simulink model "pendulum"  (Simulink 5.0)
settings: Solver=FixedStepDiscrete  StartTime=0  StopTime=2000*Ts  FixedStep=Ts  MaxStep=0.001  RelTol=1e-3
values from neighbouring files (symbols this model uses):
  angle_K = 22/0.5    (= 44)    [pendulum_init.m]
  friction2 = 0.08    [pendulum_init.m]
  Kd = 0.00349    [pendulum_init.m]
  Kd_x = 0.2    [pendulum_init.m]
  Kp = 0.1047    [pendulum_init.m]
  Kp_x = 0.2    [pendulum_init.m]
  limit_motor = 1.1    [pendulum_init.m]
  motor_bias = -0.011    [pendulum_init.m]
  position_command = 0    [pendulum_init.m]
  POSITION_EN = 0    [pendulum_init.m]
  position_K = cm_per_rotation/400    (= 0.020375)    [pendulum_init.m]
  reset_all = 0    [pendulum_init.m]
  reset_angle = 0    [pendulum_init.m]
  reset_position = 0    [pendulum_init.m]
  reset_speed = 0    [pendulum_init.m]
  RUN = 0    [pendulum_init.m]
  slope1 = 6    [pendulum_init.m]
  slope2 = 3    [pendulum_init.m]
  speed_K = cm_per_rotation*1000/60/3    (= 45.2777777778)    [pendulum_init.m]
  trigger_voltage = 0.8    [pendulum_init.m]
undefined symbols (not defined in the file or in its folder): friction1, Ts

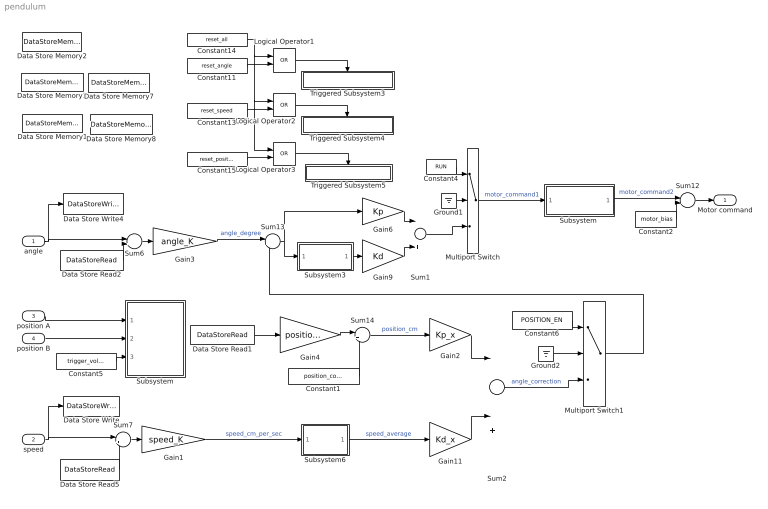
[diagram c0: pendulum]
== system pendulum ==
  angle : Inport
  speed : Inport  Port=2  ShowAdditionalParam=on
  position A : Inport  Port=3
  position B : Inport  Port=4
  Constant1 : Constant  Value=position_command  VectorParams1D=off
  Constant11 : Constant  Value=reset_angle  VectorParams1D=off
  Constant13 : Constant  Value=reset_speed  VectorParams1D=off
  Constant14 : Constant  Value=reset_all  VectorParams1D=off
  Constant15 : Constant  Value=reset_position  VectorParams1D=off
  Constant2 : Constant  Value=motor_bias  VectorParams1D=off
  Constant4 : Constant  Value=RUN  VectorParams1D=off
  Constant5 : Constant  Value=trigger_voltage  VectorParams1D=off
  Constant6 : Constant  Value=POSITION_EN  VectorParams1D=off
  Data Store Memory1 : DataStoreMemory  DataStoreName=speed_V  InitialValue=0
  Data Store Memory2 : DataStoreMemory  DataStoreName=position_count  InitialValue=0
  Data Store Memory3 : DataStoreMemory  DataStoreName=angle_V  InitialValue=0
  Data Store Memory7 : DataStoreMemory  DataStoreName=angle_V_zero  InitialValue=2.045
  Data Store Memory8 : DataStoreMemory  DataStoreName=speed_V_zero  InitialValue=0
  Data Store Read1 : DataStoreRead  DataStoreName=position_count  SampleTime=Ts
  Data Store Read2 : DataStoreRead  DataStoreName=angle_V_zero  SampleTime=Ts
  Data Store Read5 : DataStoreRead  DataStoreName=speed_V_zero  SampleTime=Ts
  Data Store Write : DataStoreWrite  DataStoreName=speed_V  SampleTime=Ts
  Data Store Write4 : DataStoreWrite  DataStoreName=angle_V  SampleTime=Ts
  Gain1 : Gain  Gain=speed_K
  Gain11 : Gain  Gain=Kd_x
  Gain2 : Gain  Gain=Kp_x
  Gain3 : Gain  Gain=angle_K
  Gain4 : Gain  Gain=position_K
  Gain6 : Gain  Gain=Kp
  Gain9 : Gain  Gain=Kd
  Ground1 : Ground
  Ground2 : Ground
  Logical Operator1 : Logic  Operator=OR  AllPortsSameDT=off
  Logical Operator2 : Logic  Operator=OR  AllPortsSameDT=off
  Logical Operator3 : Logic  Operator=OR  AllPortsSameDT=off
  Multiport Switch : MultiPortSwitch  Inputs=2  ShowAdditionalParam=on  zeroidx=on
  Multiport Switch1 : MultiPortSwitch  Inputs=2  ShowAdditionalParam=on  zeroidx=on
  Subsystem : Subsystem
  "Subsystem " : Subsystem
  Subsystem3 : Subsystem
  Subsystem6 : Subsystem
  Sum1 : Sum  Inputs=|+|||+|
  Sum{6..7,12,14} (4 alike) : Sum  Inputs=|+-
  Sum13 : Sum  Inputs=|++
  Sum2 : Sum  Inputs=||+||||||+||
  Triggered Subsystem3 : Subsystem  TreatAsAtomicUnit=on
  Triggered Subsystem4 : Subsystem  TreatAsAtomicUnit=on
  Triggered Subsystem5 : Subsystem  TreatAsAtomicUnit=on
  Motor command : Outport
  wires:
  position A/1 -> Subsystem/1(Position port A)
  Constant4/1 -> Multiport Switch/1
  Ground1/1 -> Multiport Switch/2
  Data Store Read2/1 -> Sum6/2
  Gain3/1 -> Sum13/1  "angle_degree"
  Constant13/1 -> Logical Operator2/2
  Constant11/1 -> Logical Operator1/2
  Logical Operator1/1 -> Triggered Subsystem3/Trigger
  Logical Operator2/1 -> Triggered Subsystem4/Trigger
  Constant14/1 -> Logical Operator1/1, Logical Operator2/1, Logical Operator3/1
  Constant15/1 -> Logical Operator3/2
  Logical Operator3/1 -> Triggered Subsystem5/Trigger
  Sum6/1 -> Gain3/1
  Data Store Read1/1 -> Gain4/1
  Gain4/1 -> Sum14/1
  position B/1 -> Subsystem/2(Position port B)
  Constant5/1 -> Subsystem/3(Trigger voltage)
  Gain6/1 -> Sum1/1
  Gain9/1 -> Sum1/2
  Subsystem3/1(derivation) -> Gain9/1
  Sum14/1 -> Gain2/1  "position_cm"
  Constant1/1 -> Sum14/2
  Gain2/1 -> Sum2/1
  Sum12/1 -> Motor command/1
  Constant2/1 -> Sum12/2
  Sum1/1 -> Multiport Switch/3
  Gain1/1 -> Subsystem6/1(input)  "speed_cm_per_sec"
  Subsystem6/1(filter) -> Gain11/1  "speed_average"
  Gain11/1 -> Sum2/2
  "Subsystem "/1(discontinuity) -> Sum12/1  "motor_command2"
  Multiport Switch/1 -> "Subsystem "/1(input)  "motor_command1"
  Data Store Read5/1 -> Sum7/2
  Sum7/1 -> Gain1/1
  angle/1 -> Data Store Write4/1, Sum6/1
  speed/1 -> Sum7/1, Data Store Write/1
  Ground2/1 -> Multiport Switch1/2
  Constant6/1 -> Multiport Switch1/1
  Sum2/1 -> Multiport Switch1/3  "angle_correction"
  Multiport Switch1/1 -> Sum13/2
  Sum13/1 -> Subsystem3/1(input), Gain6/1

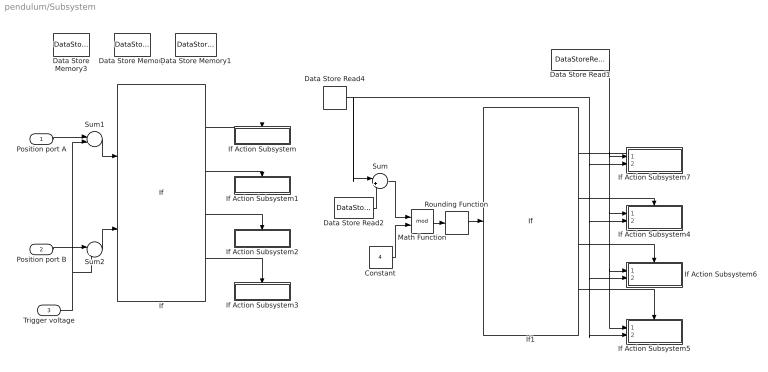
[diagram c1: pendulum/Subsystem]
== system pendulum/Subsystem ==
  Position port A : Inport
  Position port B : Inport  Port=2
  Trigger voltage : Inport  Port=3
  Constant : Constant  Value=4  ShowAdditionalParam=on
  Data Store Memory : DataStoreMemory  DataStoreName=last_state  InitialValue=3
  Data Store Memory1 : DataStoreMemory  DataStoreName=direction  InitialValue=0
  Data Store Memory3 : DataStoreMemory  DataStoreName=state  InitialValue=0
  Data Store Read1 : DataStoreRead  DataStoreName=position_count  SampleTime=Ts
  Data Store Read2 : DataStoreRead  DataStoreName=last_state  SampleTime=Ts
  Data Store Read4 : DataStoreRead  DataStoreName=state  SampleTime=Ts
  If : If  NumInputs=2  IfExpression=u1<0 & u2<0  ElseIfExpressions=u1<0 & u2>=0,u1>=0 & u2>=0,u1>=0 & u2<0  ShowElse=off
  If Action Subsystem : Subsystem  TreatAsAtomicUnit=on
  If Action Subsystem1 : Subsystem  TreatAsAtomicUnit=on
  If Action Subsystem2 : Subsystem  TreatAsAtomicUnit=on
  If Action Subsystem3 : Subsystem  TreatAsAtomicUnit=on
  If Action Subsystem4 : Subsystem  TreatAsAtomicUnit=on
  If Action Subsystem5 : Subsystem  TreatAsAtomicUnit=on
  If Action Subsystem6 : Subsystem  TreatAsAtomicUnit=on
  If Action Subsystem7 : Subsystem  TreatAsAtomicUnit=on
  If1 : If  IfExpression=u1==0  ElseIfExpressions=u1==1,u1==2,u1==3  ShowElse=off
  Math Function : Math  Operator=mod
  Rounding Function : Rounding  Operator=round
  Sum : Sum  Inputs=|+-
  Sum1 : Sum  Inputs=|+-
  Sum2 : Sum  Inputs=|+-
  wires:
  Sum/1 -> Math Function/1
  Constant/1 -> Math Function/2
  Data Store Read1/1 -> If Action Subsystem4/1(In1), If Action Subsystem5/1(In1), If Action Subsystem6/1(In1), If Action Subsystem7/1(In1)
  If1/4 -> If Action Subsystem5/Action
  If1/3 -> If Action Subsystem6/Action
  If1/2 -> If Action Subsystem4/Action
  If1/1 -> If Action Subsystem7/Action
  Data Store Read2/1 -> Sum/2
  Data Store Read4/1 -> Sum/1, If Action Subsystem6/2(In2), If Action Subsystem5/2(In2), If Action Subsystem4/2(In2), If Action Subsystem7/2(In2)
  Math Function/1 -> Rounding Function/1
  Rounding Function/1 -> If1/1
  If/4 -> If Action Subsystem3/Action
  If/3 -> If Action Subsystem2/Action
  If/2 -> If Action Subsystem1/Action
  If/1 -> If Action Subsystem/Action
  Sum1/1 -> If/1
  Sum2/1 -> If/2
  Position port A/1 -> Sum1/1
  Position port B/1 -> Sum2/1
  Trigger voltage/1 -> Sum2/2, Sum1/2

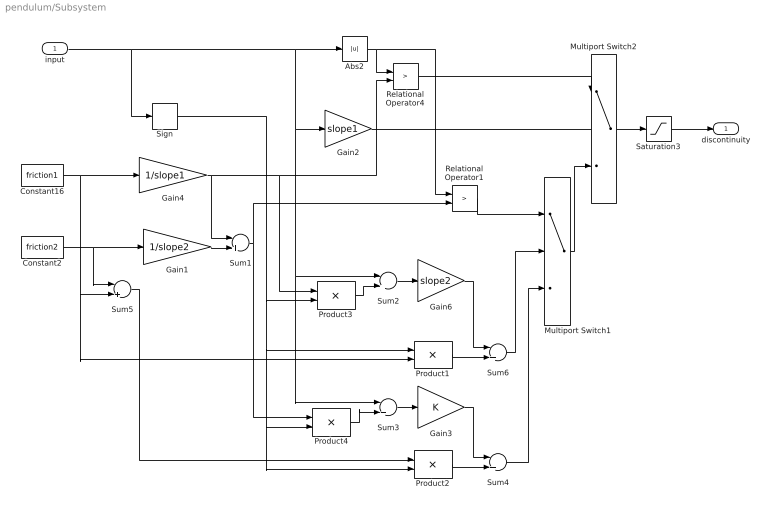
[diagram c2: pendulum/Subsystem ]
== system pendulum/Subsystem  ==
  input : Inport
  Abs2 : Abs
  Constant16 : Constant  Value=friction1  VectorParams1D=off
  Constant2 : Constant  Value=friction2  VectorParams1D=off
  Gain1 : Gain  Gain=1/slope2
  Gain2 : Gain  Gain=slope1
  Gain3 : Gain
  Gain4 : Gain  Gain=1/slope1
  Gain6 : Gain  Gain=slope2
  Multiport Switch1 : MultiPortSwitch  Inputs=2  ShowAdditionalParam=on  zeroidx=on
  Multiport Switch2 : MultiPortSwitch  Inputs=2  ShowAdditionalParam=on  zeroidx=on
  Product{1..4} (4 alike) : Product
  Relational Operator1 : RelationalOperator  Operator=>
  Relational Operator4 : RelationalOperator  Operator=>
  Saturation3 : Saturate  UpperLimit=limit_motor  LowerLimit=-limit_motor
  Sign : Signum
  Sum{1,4..6} (4 alike) : Sum  Inputs=|+|+|
  Sum2 : Sum  Inputs=|+|-|
  Sum3 : Sum  Inputs=|+|-|
  discontinuity : Outport
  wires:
  input/1 -> Sign/1, Abs2/1, Gain2/1, Sum2/1, Sum3/1
  Abs2/1 -> Relational Operator4/1, Relational Operator1/1
  Relational Operator4/1 -> Multiport Switch2/1
  Constant16/1 -> Gain4/1, Product1/2, Sum5/2
  Gain2/1 -> Multiport Switch2/2
  Constant2/1 -> Gain1/1, Sum5/1
  Gain4/1 -> Sum1/1, Relational Operator4/2, Product3/1
  Gain1/1 -> Sum1/2
  Relational Operator1/1 -> Multiport Switch1/1
  Sum1/1 -> Relational Operator1/2, Product4/1
  Sign/1 -> Product3/2, Product1/1, Product2/2, Product4/2
  Gain6/1 -> Sum6/1
  Sum2/1 -> Gain6/1
  Product3/1 -> Sum2/2
  Sum6/1 -> Multiport Switch1/2
  Product1/1 -> Sum6/2
  Gain3/1 -> Sum4/1
  Sum3/1 -> Gain3/1
  Product4/1 -> Sum3/2
  Product2/1 -> Sum4/2
  Sum5/1 -> Product2/1
  Sum4/1 -> Multiport Switch1/3
  Multiport Switch1/1 -> Multiport Switch2/3
  Multiport Switch2/1 -> Saturation3/1
  Saturation3/1 -> discontinuity/1

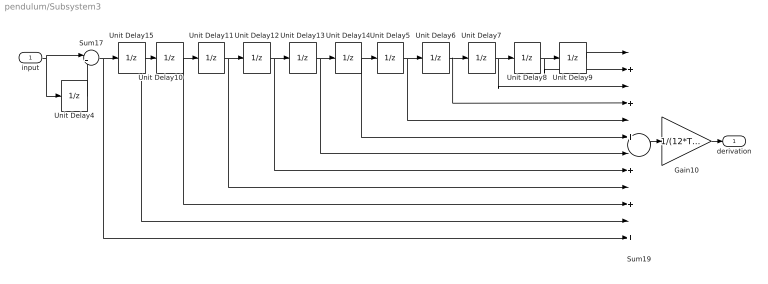
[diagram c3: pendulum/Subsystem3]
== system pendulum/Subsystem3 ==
  input : Inport
  Gain10 : Gain  Gain=1/(12*Ts)
  Sum17 : Sum  Inputs=|+-
  Sum19 : Sum  Inputs=|+|+|+|+|+|+|+|+|+|+|+|+|
  Unit Delay{4..15} (12 alike) : UnitDelay  SampleTime=Ts
  derivation : Outport
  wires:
  Gain10/1 -> derivation/1
  Sum19/1 -> Gain10/1
  Sum17/1 -> Sum19/12, Unit Delay15/1
  Unit Delay15/1 -> Sum19/11, Unit Delay10/1
  Unit Delay14/1 -> Sum19/6, Unit Delay5/1
  Unit Delay13/1 -> Sum19/7, Unit Delay14/1
  Unit Delay11/1 -> Sum19/9, Unit Delay12/1
  Unit Delay12/1 -> Sum19/8, Unit Delay13/1
  Unit Delay10/1 -> Sum19/10, Unit Delay11/1
  Unit Delay9/1 -> Sum19/1
  Unit Delay8/1 -> Sum19/2, Unit Delay9/1
  Unit Delay6/1 -> Sum19/4, Unit Delay7/1
  Unit Delay7/1 -> Sum19/3, Unit Delay8/1
  Unit Delay5/1 -> Sum19/5, Unit Delay6/1
  Unit Delay4/1 -> Sum17/2
  input/1 -> Unit Delay4/1, Sum17/1

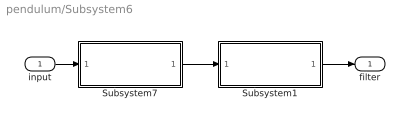
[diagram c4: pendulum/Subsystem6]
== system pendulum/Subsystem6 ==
  input : Inport
  Subsystem1 : Subsystem
  Subsystem7 : Subsystem
  filter : Outport
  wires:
  input/1 -> Subsystem7/1(input)
  Subsystem7/1(filter) -> Subsystem1/1(input)
  Subsystem1/1(filter) -> filter/1

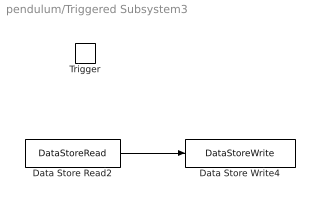
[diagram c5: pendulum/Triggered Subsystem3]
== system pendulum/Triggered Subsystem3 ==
  Trigger : TriggerPort
  Data Store Read2 : DataStoreRead  DataStoreName=angle_V  SampleTime=-1
  Data Store Write4 : DataStoreWrite  DataStoreName=angle_V_zero  SampleTime=-1
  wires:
  Data Store Read2/1 -> Data Store Write4/1

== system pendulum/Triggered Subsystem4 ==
  Trigger : TriggerPort
  Data Store Read2 : DataStoreRead  DataStoreName=speed_V  SampleTime=-1
  Data Store Write4 : DataStoreWrite  DataStoreName=speed_V_zero  SampleTime=-1
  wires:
  Data Store Read2/1 -> Data Store Write4/1

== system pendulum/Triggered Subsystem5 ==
  Trigger : TriggerPort
  Constant : Constant  Value=0
  Data Store Write3 : DataStoreWrite  DataStoreName=position_count  SampleTime=-1
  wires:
  Constant/1 -> Data Store Write3/1

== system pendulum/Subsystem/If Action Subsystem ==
  Action Port : ActionPort  ActionType=then
  Constant : Constant  Value=0
  Data Store Write : DataStoreWrite  DataStoreName=state  SampleTime=-1
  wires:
  Constant/1 -> Data Store Write/1

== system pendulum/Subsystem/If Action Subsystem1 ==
  Action Port : ActionPort  ActionType=elseif
  Constant : Constant
  Data Store Write : DataStoreWrite  DataStoreName=state  SampleTime=-1
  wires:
  Constant/1 -> Data Store Write/1

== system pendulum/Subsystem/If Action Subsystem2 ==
  Action Port : ActionPort  ActionType=elseif
  Constant : Constant  Value=2
  Data Store Write : DataStoreWrite  DataStoreName=state  SampleTime=-1
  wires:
  Constant/1 -> Data Store Write/1

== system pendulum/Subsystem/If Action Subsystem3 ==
  Action Port : ActionPort  ActionType=elseif
  Constant : Constant  Value=3
  Data Store Write : DataStoreWrite  DataStoreName=state  SampleTime=-1
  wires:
  Constant/1 -> Data Store Write/1

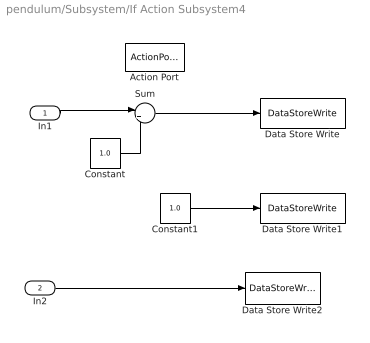
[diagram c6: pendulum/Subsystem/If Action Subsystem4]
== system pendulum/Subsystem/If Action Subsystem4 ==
  In1 : Inport
  In2 : Inport  Port=2
  Action Port : ActionPort  InitializeStates=reset  ActionType=elseif
  Constant : Constant  Value=1.0
  Constant1 : Constant  Value=1.0
  Data Store Write : DataStoreWrite  DataStoreName=position_count  SampleTime=-1
  Data Store Write1 : DataStoreWrite  DataStoreName=direction  SampleTime=Ts
  Data Store Write2 : DataStoreWrite  DataStoreName=last_state  SampleTime=-1
  Sum : Sum  Inputs=|++
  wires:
  In1/1 -> Sum/1
  Sum/1 -> Data Store Write/1
  Constant/1 -> Sum/2
  Constant1/1 -> Data Store Write1/1
  In2/1 -> Data Store Write2/1

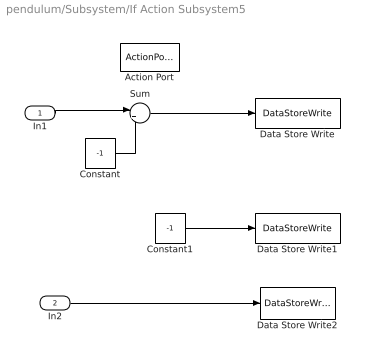
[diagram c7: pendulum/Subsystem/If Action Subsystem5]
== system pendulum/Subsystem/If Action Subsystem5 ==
  In1 : Inport
  In2 : Inport  Port=2
  Action Port : ActionPort  InitializeStates=reset  ActionType=elseif
  Constant : Constant  Value=-1
  Constant1 : Constant  Value=-1
  Data Store Write : DataStoreWrite  DataStoreName=position_count  SampleTime=-1
  Data Store Write1 : DataStoreWrite  DataStoreName=direction  SampleTime=Ts
  Data Store Write2 : DataStoreWrite  DataStoreName=last_state  SampleTime=-1
  Sum : Sum  Inputs=|++
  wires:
  Constant1/1 -> Data Store Write1/1
  Constant/1 -> Sum/2
  Sum/1 -> Data Store Write/1
  In1/1 -> Sum/1
  In2/1 -> Data Store Write2/1

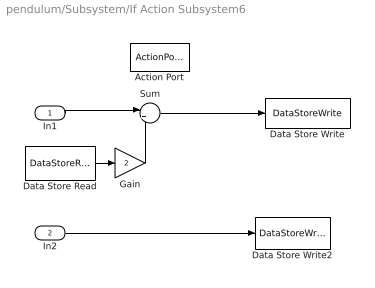
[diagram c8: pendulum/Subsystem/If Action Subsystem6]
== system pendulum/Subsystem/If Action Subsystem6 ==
  In1 : Inport
  In2 : Inport  Port=2
  Action Port : ActionPort  InitializeStates=reset  ActionType=elseif
  Data Store Read : DataStoreRead  DataStoreName=direction  SampleTime=Ts
  Data Store Write : DataStoreWrite  DataStoreName=position_count  SampleTime=-1
  Data Store Write2 : DataStoreWrite  DataStoreName=last_state  SampleTime=-1
  Gain : Gain  Gain=2
  Sum : Sum  Inputs=|++
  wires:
  In1/1 -> Sum/1
  Sum/1 -> Data Store Write/1
  Data Store Read/1 -> Gain/1
  Gain/1 -> Sum/2
  In2/1 -> Data Store Write2/1

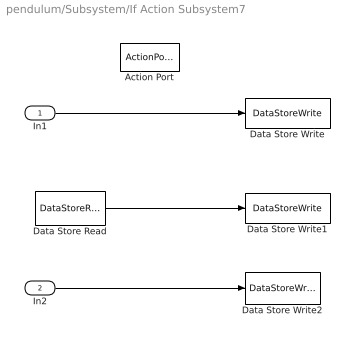
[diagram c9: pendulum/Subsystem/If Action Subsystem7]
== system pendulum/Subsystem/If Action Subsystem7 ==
  In1 : Inport
  In2 : Inport  Port=2
  Action Port : ActionPort  InitializeStates=reset  ActionType=then
  Data Store Read : DataStoreRead  DataStoreName=direction  SampleTime=Ts
  Data Store Write : DataStoreWrite  DataStoreName=position_count  SampleTime=-1
  Data Store Write1 : DataStoreWrite  DataStoreName=direction  SampleTime=Ts
  Data Store Write2 : DataStoreWrite  DataStoreName=last_state  SampleTime=-1
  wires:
  In2/1 -> Data Store Write2/1
  Data Store Read/1 -> Data Store Write1/1
  In1/1 -> Data Store Write/1

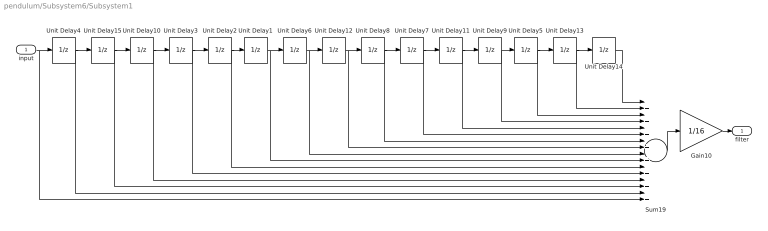
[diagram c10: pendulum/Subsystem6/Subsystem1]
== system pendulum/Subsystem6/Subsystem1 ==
  input : Inport
  Gain10 : Gain  Gain=1/16
  Sum19 : Sum  Inputs=|+|+|+|+|+|+|+|+|+|+|+|+|+|+|+|+|
  Unit Delay{1..15} (15 alike) : UnitDelay  SampleTime=Ts
  filter : Outport
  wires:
  input/1 -> Unit Delay4/1, Sum19/16
  Unit Delay4/1 -> Unit Delay15/1, Sum19/15
  Unit Delay15/1 -> Unit Delay10/1, Sum19/14
  Unit Delay10/1 -> Unit Delay3/1, Sum19/13
  Unit Delay3/1 -> Unit Delay2/1, Sum19/12
  Unit Delay2/1 -> Unit Delay1/1, Sum19/11
  Unit Delay1/1 -> Unit Delay6/1, Sum19/10
  Unit Delay6/1 -> Unit Delay12/1, Sum19/9
  Unit Delay12/1 -> Unit Delay8/1, Sum19/8
  Unit Delay8/1 -> Unit Delay7/1, Sum19/7
  Unit Delay7/1 -> Unit Delay11/1, Sum19/6
  Unit Delay11/1 -> Unit Delay9/1, Sum19/5
  Unit Delay9/1 -> Unit Delay5/1, Sum19/4
  Unit Delay5/1 -> Unit Delay13/1, Sum19/3
  Unit Delay13/1 -> Unit Delay14/1, Sum19/2
  Unit Delay14/1 -> Sum19/1
  Sum19/1 -> Gain10/1
  Gain10/1 -> filter/1

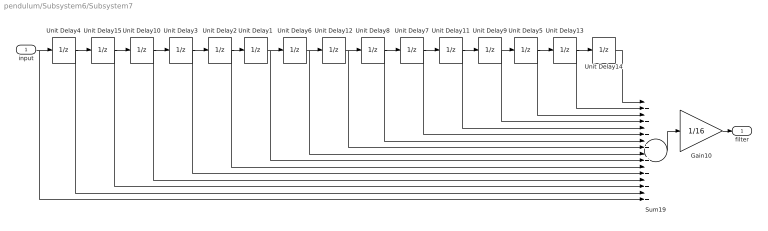
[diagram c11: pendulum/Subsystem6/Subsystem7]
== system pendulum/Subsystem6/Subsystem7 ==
  input : Inport
  Gain10 : Gain  Gain=1/16
  Sum19 : Sum  Inputs=|+|+|+|+|+|+|+|+|+|+|+|+|+|+|+|+|
  Unit Delay{1..15} (15 alike) : UnitDelay  SampleTime=Ts
  filter : Outport
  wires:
  Gain10/1 -> filter/1
  Sum19/1 -> Gain10/1
  Unit Delay14/1 -> Sum19/1
  Unit Delay13/1 -> Sum19/2, Unit Delay14/1
  Unit Delay5/1 -> Sum19/3, Unit Delay13/1
  Unit Delay9/1 -> Sum19/4, Unit Delay5/1
  Unit Delay11/1 -> Sum19/5, Unit Delay9/1
  Unit Delay7/1 -> Sum19/6, Unit Delay11/1
  Unit Delay8/1 -> Sum19/7, Unit Delay7/1
  Unit Delay12/1 -> Sum19/8, Unit Delay8/1
  Unit Delay6/1 -> Sum19/9, Unit Delay12/1
  Unit Delay1/1 -> Sum19/10, Unit Delay6/1
  Unit Delay2/1 -> Sum19/11, Unit Delay1/1
  Unit Delay3/1 -> Sum19/12, Unit Delay2/1
  Unit Delay10/1 -> Sum19/13, Unit Delay3/1
  Unit Delay15/1 -> Sum19/14, Unit Delay10/1
  Unit Delay4/1 -> Sum19/15, Unit Delay15/1
  input/1 -> Sum19/16, Unit Delay4/1
